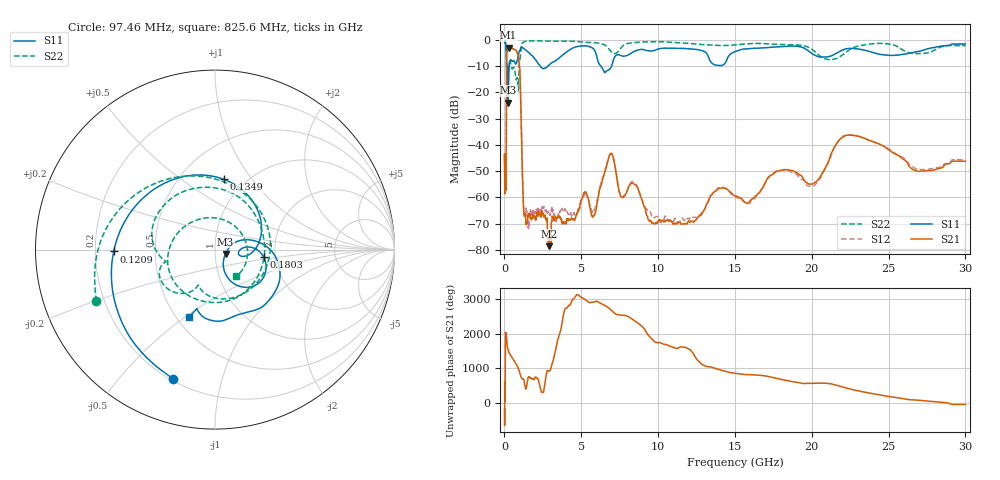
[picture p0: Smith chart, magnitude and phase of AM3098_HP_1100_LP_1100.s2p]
! Date/Time: Thu, Feb 28, 2019 8:44 AM
! Network Analyzer: Agilent Technologies E8364B Rev: A.07.50.67
! Sweep from 0.010 to 30.000 GHz, 1601 Points, Sweep Type: LOG
! Power Supply: 5.023 V, 0.002 A
# Hz S DB R 50
!freq MagS11 AngS11 MagS21 AngS21 MagS12 AngS12 MagS22 AngS22
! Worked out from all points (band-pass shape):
!   1601 points, 10 MHz to 30 GHz, reference 50 ohm
!   highest |S21| = -3.06 dB at 266.5 MHz (marker M1); lowest = -78.5 dB at 2.884 GHz (marker M2)
!   |S21| within 3 dB of the highest: 149.2 MHz to 886.2 MHz (737 MHz wide, 142 % of centre)
!   lowest |S11| = -23.9 dB at 248.4 MHz (marker M3), VSWR 1.14, Z = 56.2 - j2.79 ohm
!   |S11| at or under -10 dB: 140.1 MHz to 311.7 MHz (171.6 MHz wide, 76 % of centre); 2.323 GHz to 2.838 GHz (515.8 MHz wide, 20 % of centre); 6.257 GHz to 6.974 GHz (716.8 MHz wide, 10.8 % of centre)
!   |S22| runs from -19.5 to -0.5 dB; largest |S21 - S12| = 0.012
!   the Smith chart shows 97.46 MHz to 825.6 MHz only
!   S11 on the Smith chart (normalised r, x): 97.46 MHz: 0.21, -0.71; 120.9 MHz: 0.28, -0.01; 134.9 MHz: 0.80, +0.74; 180.3 MHz: 1.74, -0.16; 825.6 MHz: 0.58, -0.52
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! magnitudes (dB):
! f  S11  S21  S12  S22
! 10 MHz  -0.4  -43.7  -44.8  -0.7
! 38.04 MHz  -0.4  -56.9  -58.2  -0.9
! 97.46 MHz  -2.4  -57.3  -54.6  -2.8
! 120.9 MHz  -5.0  -36.3  -36.2  -6.5
! 134.9 MHz  -8.1  -14.7  -14.6  -10.3
! 144.7 MHz  -12.2  -7.4  -7.4  -11.5
! 180.3 MHz  -11.2  -3.9  -3.9  -9.9
! 248.4 MHz  -23.9  -3.1  -3.0  -11.0
! 266.5 MHz  -18.0  -3.1  -3.0  -10.8
! 550.5 MHz  -8.1  -3.5  -3.5  -10.8
! 825.6 MHz  -8.0  -4.9  -4.9  -14.4
! 1.009 GHz  -4.1  -13.0  -13.0  -7.6
! 1.282 GHz  -3.5  -66.1  -65.8  -0.9
! 2.084 GHz  -8.1  -67.3  -65.0  -0.5
! 2.884 GHz  -9.7  -78.5  -66.3  -0.6
! 5.783 GHz  -3.4  -66.9  -65.8  -1.2
! 6.89 GHz  -10.9  -43.5  -43.4  -4.2
! 7.926 GHz  -6.1  -58.4  -58.4  -1.6
! 11.95 GHz  -3.5  -69.2  -67.9  -1.4
! 20.1 GHz  -5.6  -54.8  -55.9  -4.1
! 22.56 GHz  -3.3  -36.3  -36.2  -3.5
! 30 GHz  -1.7  -46.2  -45.7  -2.3
